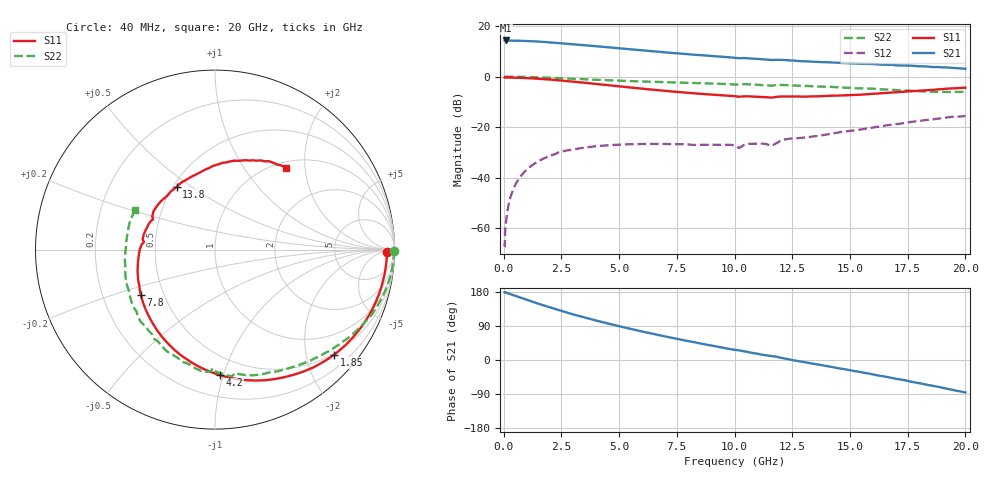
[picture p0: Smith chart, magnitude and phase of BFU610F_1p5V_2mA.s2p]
! Filename:  P:\Prog\Test\Noise\ATS_data\Testdata_Net\SplitFiles\BFU610_2W_A5_HighFreq_1.5V_2mA_D.s2p
! Date/Time: Wed 10/Aug/2011 16:54:02
! BFU610_2W_A5_HighFreq_Bias2_1.5V_1mA_10mA_R.s2p
! MDIF S-parameter v. bias file
! BFU610_2W_A5_HighFreq_1.5V_1mA_10mA
! Date/time Mon Aug 08 13:57:57 2011
! VAR V_out= 1.5000
! VAR I_out= 1.9850
! VAR V_in= 0.8709
! VAR I_in= 0.0152
! Device data file deembeded for feedlines and parallel
! Original file: \SplitFiles\BFU610_2W_A5_HighFreq_1.5V_2mA_R.s2p
! Feed-files: PR003V01_101208_Feed1.s2p, PR003V01_101208_Feed2.s2p
! Parallel-file: PR003V01_101208_Par.s2p
# MHz S MA R 50
!  Freq-MHz  S11-mag  S11-arg  S21-mag  S21-arg  S12-mag  S12-arg  S22-mag  S22-arg
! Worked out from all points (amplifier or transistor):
!   167 points, 40 MHz to 20 GHz, reference 50 ohm
!   highest |S21| = 14.3 dB at 80 MHz (marker M1)
!   |S21| within 3 dB of that: start of sweep to 4.847 GHz
!   unconditionally stable (mu >= 1): 6.606 GHz to 19.24 GHz
!   at 550 MHz: K = 0.01, MSG = 28.1 dB, |S12| = -42.0 dB
!   at 4.2 GHz: K = 0.55, MSG = 19.6 dB, |S12| = -27.4 dB
!   at 20 GHz: K = 0.97, MSG = 9.4 dB, |S12| = -15.6 dB
!   S11 on the Smith chart (normalised r, x): 40 MHz: 41, -15; 1.85 GHz: 0.47, -2.56; 4.2 GHz: 0.36, -0.98; 7.8 GHz: 0.37, -0.24; 13.8 GHz: 0.52, +0.44; 20 GHz: 1.10, +1.59
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40  0.9577 -0.9  5.18 179.1  0.0004943 83.9  0.996 -0.4
50  0.9491 -1.2  5.162 179.2  0.0004419 127.6  0.9958 -0.5
60  0.959 -1.1  5.175 178.3  0.0008323 102.6  0.9967 -0.6
80  0.9576 -1.8  5.184 178.2  0.001041 91.0  0.9968 -0.8
260  0.956 -6.0  5.164 174.3  0.003634 89.4  0.996 -2.9
550  0.9501 -12.7  5.147 168.1  0.007944 84.7  0.9926 -6.1
1300  0.9183 -29.5  4.988 152.6  0.01853 71.7  0.974 -14.2
1850  0.8848 -41.5  4.809 141.6  0.02531 63.2  0.9553 -19.7
2700  0.8178 -59.2  4.495 125.9  0.03434 51.0  0.9173 -27.7
3400  0.7633 -72.8  4.208 113.9  0.03874 43.2  0.889 -33.7
4200  0.6998 -87.7  3.91 101.1  0.04272 35.2  0.8575 -39.9
5400  0.6151 -108.8  3.486 83.4  0.04577 26.0  0.8176 -48.8
6800  0.5309 -132.3  3.059 64.7  0.04639 18.4  0.7776 -58.4
7800  0.4842 -148.7  2.815 52.2  0.04589 15.7  0.7538 -65.2
9400  0.4287 -174.0  2.483 33.4  0.04474 15.8  0.7193 -76.4
10200  0.3984 173.9  2.31 25.4  0.03868 17.2  0.6962 -80.2
12000  0.4035 148.4  2.144 6.0  0.05421 33.8  0.6836 -94.4
13400  0.4071 126.7  1.966 -9.6  0.06547 27.7  0.6422 -107.9
13800  0.4099 121.5  1.928 -13.7  0.06907 28.0  0.6317 -111.5
16800  0.4859 84.8  1.706 -47.2  0.1118 15.7  0.55 -147.7
18400  0.5398 67.3  1.573 -66.2  0.1398 3.0  0.5056 -173.7
20000  0.6034 49.3  1.427 -85.7  0.1655 -13.5  0.498 154.0
